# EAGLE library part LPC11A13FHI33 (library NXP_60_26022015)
32-bit ARM Cortex-M0 microcontroller; up to 32 kB flash, 8 kB SRAM, 4 kB EEPROM; configurable analog/mixed-signal The LPC11Axx are an ARM Cortex-M0 based, low-cost 32-bit MCU family, designed for 8/16-bit microcontroller applications, offering performance, low power, simple instruction set and memory addressing together with reduced code size compared to existing 8/16-bit architectures. The LPC11Axx operate at CPU frequencies of up to 50 MHz. Analog/mixed-signal subsystems can be configured by software from interconnected digital and analog peripherals. The digital peripherals on the LPC11Axx include up to 32 kB of flash memory, up to 4 kB of EEPROM data memory, up to 8 kB of SRAM data memory, a Fast-mode Plus I 2 C-bus interface, a RS-485/EIA-485 USART, two SSP controllers, four general purpose counter/timers, and up to 42 general purpose I/O pins. Analog peripherals include a 10-bit ADC, a 10-bit DAC, an analog comparator, a temperature sensor, an internal voltage reference, and UnderVoltage LockOut (UVLO) protection. AAL Eindhoven MK
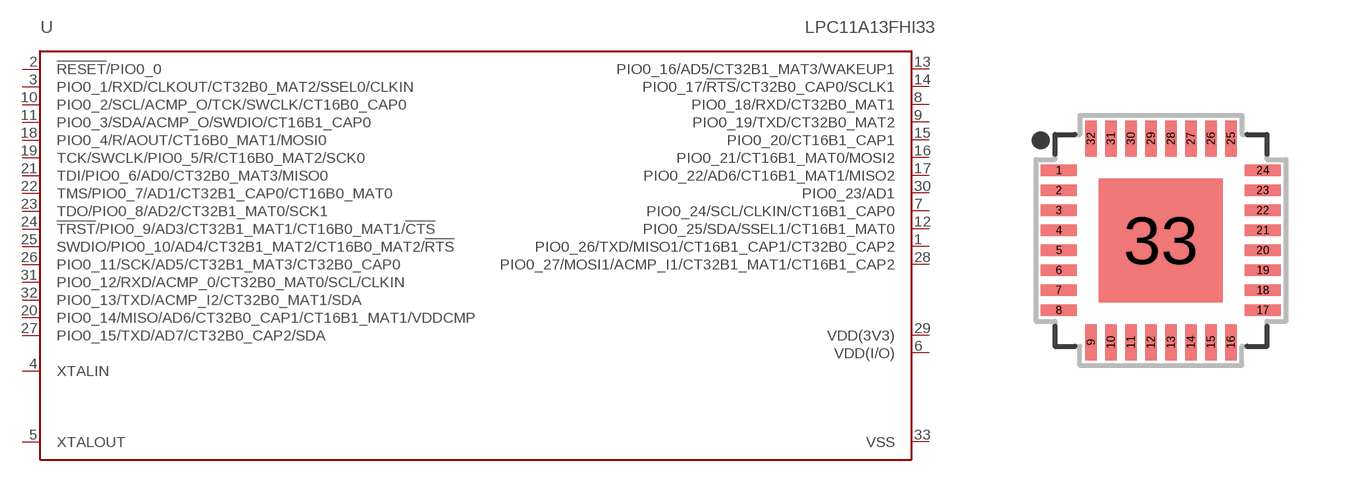
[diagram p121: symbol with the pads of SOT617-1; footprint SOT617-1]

Designator prefix U

## LPC11A13FHI33  [SOT617-1]
1  PIO0_26/TXD/MISO1/CT16B1_CAP1/CT32B0_CAP2
2  !RESET!/PIO0_0
3  PIO0_1/RXD/CLKOUT/CT32B0_MAT2/SSEL0/CLKIN
4  XTALIN  pas
5  XTALOUT  pas
6  VDD(I/O)  pwr
7  PIO0_24/SCL/CLKIN/CT16B1_CAP0
8  PIO0_18/RXD/CT32B0_MAT1
9  PIO0_19/TXD/CT32B0_MAT2
10  PIO0_2/SCL/ACMP_O/TCK/SWCLK/CT16B0_CAP0
11  PIO0_3/SDA/ACMP_O/SWDIO/CT16B1_CAP0
12  PIO0_25/SDA/SSEL1/CT16B1_MAT0
13  PIO0_16/AD5/CT32B1_MAT3/WAKEUP1
14  PIO0_17/!RTS!/CT32B0_CAP0/SCLK1
15  PIO0_20/CT16B1_CAP1
16  PIO0_21/CT16B1_MAT0/MOSI2
17  PIO0_22/AD6/CT16B1_MAT1/MISO2
18  PIO0_4/R/AOUT/CT16B0_MAT1/MOSI0
19  TCK/SWCLK/PIO0_5/R/CT16B0_MAT2/SCK0
20  PIO0_14/MISO/AD6/CT32B0_CAP1/CT16B1_MAT1/VDDCMP
21  TDI/PIO0_6/AD0/CT32B0_MAT3/MISO0
22  TMS/PIO0_7/AD1/CT32B1_CAP0/CT16B0_MAT0
23  TDO/PIO0_8/AD2/CT32B1_MAT0/SCK1
24  !TRST!/PIO0_9/AD3/CT32B1_MAT1/CT16B0_MAT1/!CTS!
25  SWDIO/PIO0_10/AD4/CT32B1_MAT2/CT16B0_MAT2/!RTS!
26  PIO0_11/SCK/AD5/CT32B1_MAT3/CT32B0_CAP0
27  PIO0_15/TXD/AD7/CT32B0_CAP2/SDA
28  PIO0_27/MOSI1/ACMP_I1/CT32B1_MAT1/CT16B1_CAP2
29  VDD(3V3)  pwr
30  PIO0_23/AD1
31  PIO0_12/RXD/ACMP_0/CT32B0_MAT0/SCL/CLKIN
32  PIO0_13/TXD/ACMP_I2/CT32B0_MAT1/SDA
33  VSS  pwr

## Footprint SOT617-1 (pad centres in mm)
SOT617-1 HVQFN32: plastic thermal enhanced very thin quad flat package; no leads; 32 terminals; body 5 x 5 x 0.85 mm JEDEC: MO-220 IEC: ---
smd 0.9 x 0.29: 1 -2.55,1.75; 2 -2.55,1.25; 3 -2.55,0.75; 4 -2.55,0.25; 5 -2.55,-0.25; 6 -2.55,-0.75; 7 -2.55,-1.25; 8 -2.55,-1.75; 17 2.55,-1.75; 18 2.55,-1.25; 19 2.55,-0.75; 20 2.55,-0.25; 21 2.55,0.25; 22 2.55,0.75; 23 2.55,1.25; 24 2.55,1.75
smd 0.29 x 0.9: 9 -1.75,-2.55; 10 -1.25,-2.55; 11 -0.75,-2.55; 12 -0.25,-2.55; 13 0.25,-2.55; 14 0.75,-2.55; 15 1.25,-2.55; 16 1.75,-2.55; 25 1.75,2.55; 26 1.25,2.55; 27 0.75,2.55; 28 0.25,2.55; 29 -0.25,2.55; 30 -0.75,2.55; 31 -1.25,2.55; 32 -1.75,2.55
smd 3.1 x 3.1: 33 0,0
